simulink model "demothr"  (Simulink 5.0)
settings: Solver=ode45  StartTime=0.0  StopTime=200  RelTol=1e-3
libraries: MarineGNC x5, simulink x2, simulink_extras x2

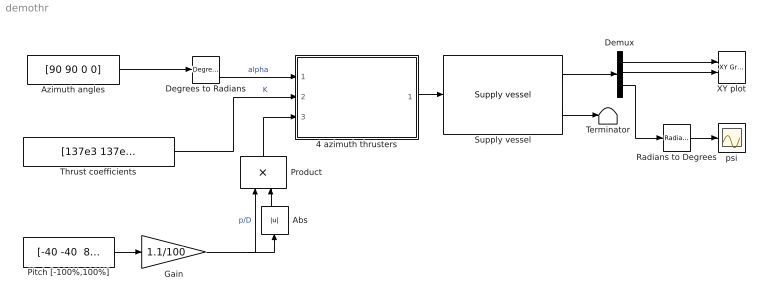
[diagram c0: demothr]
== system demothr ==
  4 azimuth thrusters : Subsystem
  Abs : Abs  Orientation=up
  Azimuth angles : Constant  Value=[90 90 0 0]
  Degrees to Radians : simulink_extras/Transformations/Degrees to Radians
  Demux : Demux  Outputs=3
  Gain : Gain  Gain=1.1/100
  Pitch [-100%,100%] : Constant  Value="[-40 -40  80 80]"
  Product : Product  Orientation=up
  Radians to Degrees : simulink_extras/Transformations/Radians to Degrees
  Supply vessel : MarineGNC/Models/Vessels/Supply vessel  D=[5.0242e4 0 0; 0 2.7229e5 -4.3933e6; 0 -4.3933e6 4.1894e8]  Minv=inv( [5.3122e6 0 0; 0 8.2831e6 0; 0 0 3.7454e9] )
  Terminator : Terminator
  Thrust coefficients : Constant  Value=[137e3 137e3 137e3 137e3]
  XY plot : simulink/Sinks/XY Graph  xmin=-500  xmax=500  ymin=-500  ymax=500  st=-1
  psi : Scope
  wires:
  4 azimuth thrusters/1(tau) -> Supply vessel/1
  Supply vessel/1 -> Demux/1
  Demux/1 -> XY plot/1
  Demux/2 -> XY plot/2
  Supply vessel/2 -> Terminator/1
  Degrees to Radians/1 -> 4 azimuth thrusters/1(alpha)  "alpha"
  Thrust coefficients/1 -> 4 azimuth thrusters/2(K(n))  "K"
  Pitch [-100%,100%]/1 -> Gain/1
  Abs/1 -> Product/2
  Gain/1 -> Product/1, Abs/1  "p/D"
  Product/1 -> 4 azimuth thrusters/3(u)
  Demux/3 -> Radians to Degrees/1
  Radians to Degrees/1 -> psi/1
  Azimuth angles/1 -> Degrees to Radians/1

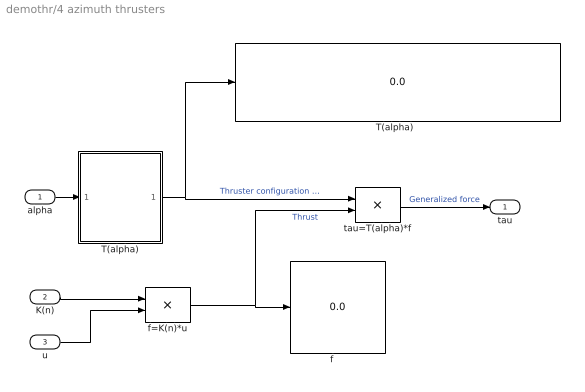
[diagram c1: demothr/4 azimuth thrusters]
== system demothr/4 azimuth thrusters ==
  alpha : Inport
  K(n) : Inport  Port=2
  u : Inport  Port=3
  T(alpha) : Subsystem
  "T(alpha)  " : Display
  "f    " : Display
  f=K(n)*u : Product
  tau=T(alpha)*f : Product  Multiplication=Matrix(*)
  tau : Outport
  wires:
  f=K(n)*u/1 -> "f    "/1, tau=T(alpha)*f/2  "Thrust"
  u/1 -> f=K(n)*u/2
  K(n)/1 -> f=K(n)*u/1
  tau=T(alpha)*f/1 -> tau/1  "Generalized force"
  alpha/1 -> T(alpha)/1(alpha)
  T(alpha)/1(T) -> "T(alpha)  "/1, tau=T(alpha)*f/1  "Thruster configuration matrix"

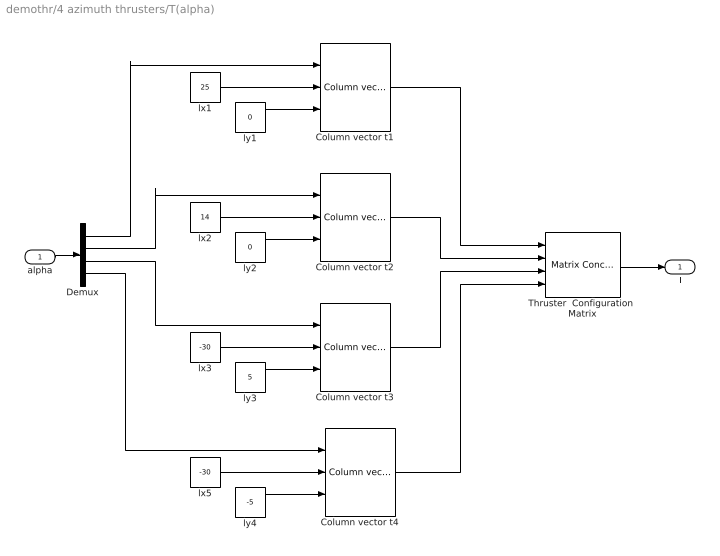
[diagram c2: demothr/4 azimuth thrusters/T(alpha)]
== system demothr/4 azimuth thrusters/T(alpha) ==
  alpha : Inport
  Column vector t{1..4} (4 alike) : MarineGNC/Models/Actuators/Column vector t1  SimViewingDevice=off  DataTypeOverride=UseLocalSettings  MinMaxOverflowLogging=UseLocalSettings
  Demux : Demux
  Thruster  Configuration  Matrix : simulink/Math Operations/Matrix Concatenation  numInports=4  catMethod=Horizontal
  lx1 : Constant  Value=25
  lx2 : Constant  Value=14
  lx3 : Constant  Value=-30
  lx5 : Constant  Value=-30
  ly1 : Constant  Value=0
  ly2 : Constant  Value=0
  ly3 : Constant  Value=5
  ly4 : Constant  Value=-5
  T : Outport
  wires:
  ly4/1 -> Column vector t4/3
  lx5/1 -> Column vector t4/2
  ly3/1 -> Column vector t3/3
  lx3/1 -> Column vector t3/2
  ly2/1 -> Column vector t2/3
  lx2/1 -> Column vector t2/2
  ly1/1 -> Column vector t1/3
  lx1/1 -> Column vector t1/2
  Thruster  Configuration  Matrix/1 -> T/1
  alpha/1 -> Demux/1
  Demux/4 -> Column vector t4/1
  Demux/3 -> Column vector t3/1
  Demux/2 -> Column vector t2/1
  Demux/1 -> Column vector t1/1
  Column vector t4/1 -> Thruster  Configuration  Matrix/4
  Column vector t3/1 -> Thruster  Configuration  Matrix/3
  Column vector t2/1 -> Thruster  Configuration  Matrix/2
  Column vector t1/1 -> Thruster  Configuration  Matrix/1
